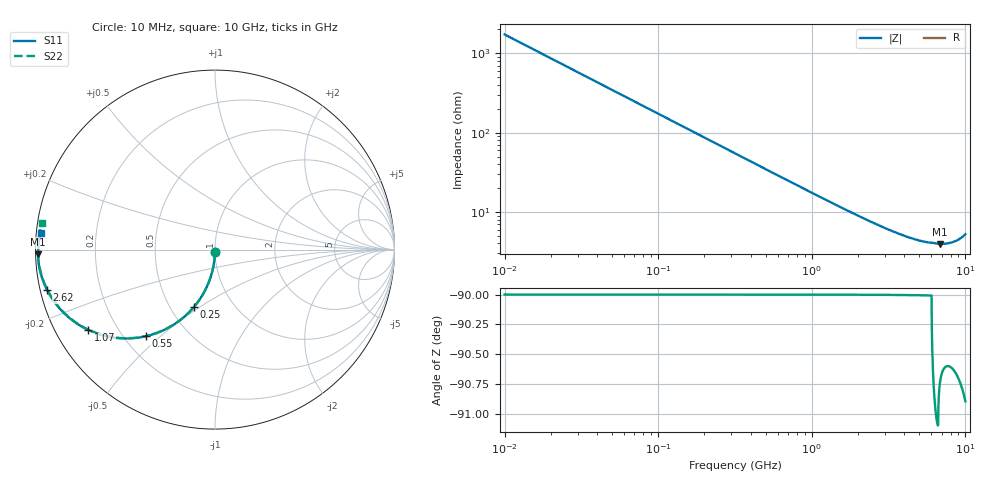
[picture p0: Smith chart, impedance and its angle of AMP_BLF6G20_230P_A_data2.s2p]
! Created Tue Mar 23 14:44:52 2010
# ghz S ma R 50
! 2 Port Network Data from SP1.SP block
! freq  magS11  angS11  magS21  angS21  magS12  angS12  magS22  angS22
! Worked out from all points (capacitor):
!   1000 points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, 10 MHz to 10 GHz, reference 50 ohm
!   read as one part in shunt: C = 9.2 pF near 60 MHz
!   lowest |Z| = 3.95 ohm at 6.85 GHz (marker M1)
!   S11 on the Smith chart (normalised r, x): 10 MHz: 1.00, -0.03; 250 MHz: 0.66, -0.47; 550 MHz: 0.29, -0.45; 1.07 GHz: 0.10, -0.29; 2.62 GHz: 0.02, -0.12; 10 GHz: 0.01, +0.05
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0.01  0.01437 -90.8  0.9999 -0.8  0.9999 -0.8  0.01437 -90.8
0.04  0.05739 -93.3  0.9984 -3.3  0.9984 -3.3  0.05739 -93.3
0.07  0.1001 -95.8  0.995 -5.8  0.995 -5.8  0.1001 -95.8
0.08  0.1142 -96.6  0.9935 -6.6  0.9935 -6.6  0.1142 -96.6
0.1  0.1422 -98.3  0.9898 -8.3  0.9898 -8.3  0.1422 -98.3
0.13  0.1836 -100.7  0.983 -10.7  0.983 -10.7  0.1836 -100.7
0.16  0.224 -103.1  0.9746 -13.1  0.9746 -13.1  0.224 -103.1
0.2  0.2761 -106.2  0.9611 -16.2  0.9611 -16.2  0.2761 -106.2
0.25  0.3379 -109.9  0.9412 -20.0  0.9412 -20.0  0.3379 -110.0
0.38  0.4787 -118.9  0.878 -28.9  0.878 -28.9  0.4787 -119.0
0.55  0.6189 -128.7  0.7854 -38.7  0.7854 -38.7  0.6189 -128.8
0.8  0.7525 -139.5  0.6586 -49.5  0.6586 -49.5  0.7525 -139.6
1.07  0.8356 -147.5  0.5493 -57.7  0.5493 -57.7  0.8356 -147.8
1.35  0.8856 -153.4  0.4644 -63.6  0.4644 -63.6  0.8856 -153.7
1.68  0.9203 -158.4  0.3913 -68.5  0.3913 -68.5  0.9203 -158.7
2.62  0.9623 -166.4  0.2721 -76.7  0.2721 -76.7  0.9623 -167.0
3.34  0.9744 -169.9  0.2247 -80.3  0.2247 -80.3  0.9744 -170.7
5.01  0.9849 -174.9  0.1728 -85.5  0.1728 -85.5  0.9849 -176.1
6.67  0.9855 -178.1  0.1567 -89.9  0.1567 -89.9  0.9845 -179.8
6.85  0.986 -178.5  0.1567 -90.1  0.1567 -90.1  0.9852 179.8
8.34  0.9846 178.7  0.1659 -93.1  0.1659 -93.1  0.9839 176.4
10  0.9758 174.7  0.2061 -97.9  0.2061 -97.9  0.9747 171.2
